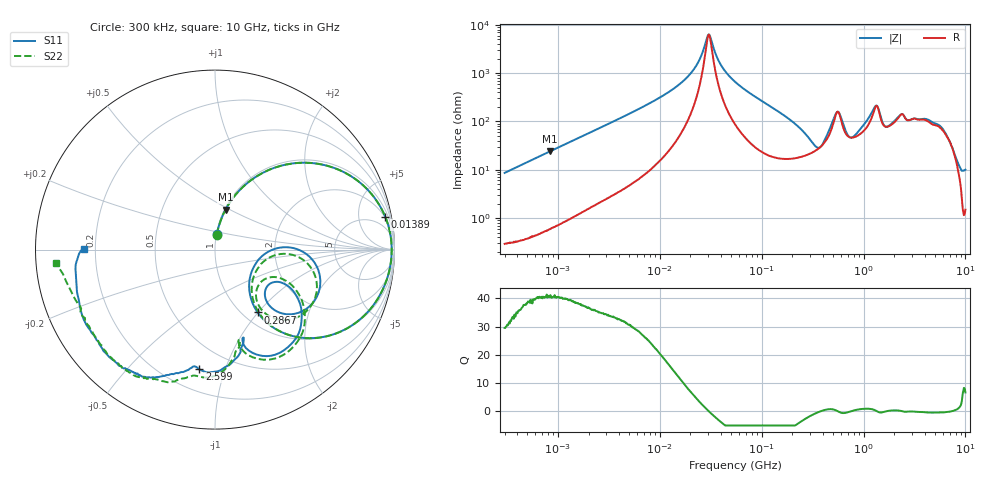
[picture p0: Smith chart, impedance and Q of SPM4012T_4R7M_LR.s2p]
! S-Parameter Data Generated by TDK Corporation
! Copyright(C) 2019 TDK Corporation.
! All Rights Reserved.
! TDK P/N: SPM4012T-4R7M-LR (Inductor)
! Property: L=4.7uH at 100kHz
! Size(LxWxT): 4.4x4.1x1.2mm
! Model Type: s2p (Touchstone File Format Version 1.0)
! Frequency: DC=Yes Start=0.3MHz Stop=10000MHz 802points Log-sweep
! Model Generated on Sep. 23, 2019
! Port Assignments:
!  1 ---@@@--- 2
! Applicable Conditions:
!  Temperature = 25 degC
!  DC Bias Current = 0 A
!  Small Signal Operation
! Terms and conditions regarding TDK Simulation Models
! (1)This simulation model is being provided solely for informational purposes. Please refer to the specifications of the products in terms of detailed characteristics of such products.
! (2)In no event shall TDK Corporation of any of its subsidiaries be liable for any loss or damage arising, directly or indirectly,
!  From any information contained in this simulation model, including, but not limited to loss or damages arising from any inaccuracies, omissions or errors in connection with such information.
! (3)Any and all copyrights on this simulation model are owned by TDK Corporation.
!  Duplication or redistribution of this simulation model without prior written permission from TDK Corporation is prohibited.
! (4)This simulation model is subject to any modification or change without any prior notice.
! (5)Neither TDK Corporation nor any of its subsidiaries shall make any warranty, express or implied,
!  Including but not limited to the correctness, implied warranties of merchantability and fitness for a particular purpose with respect to this simulation models.
! (6)The use of this simulation model shall be deemed to have consented to the terms and conditions hereof.
# Hz S MA R 50
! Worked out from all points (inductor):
!   801 points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, 300 kHz to 10 GHz, reference 50 ohm
!   read as one part in series: L = 4.57 uH near 318.3 kHz
!   highest Q = 40.6 at 832.9 kHz (marker M1), where L = 4.57 uH
!   self-resonance near 30.31 MHz
!   S11 on the Smith chart (normalised r, x): 300 kHz: 1.01, +0.17; 13.89 MHz: 2, +10; 286.7 MHz: 1.17, -0.99; 2.599 GHz: 0.34, -0.82; 10 GHz: 0.16, +0.00
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300000  0.08476 83.1  0.9935 -5.0  0.9935 -4.9  0.08438 83.1
832928  0.2309 75.2  0.9672 -13.4  0.9675 -13.4  0.2307 75.2
1713600  0.4349 62.6  0.8888 -25.8  0.8891 -25.8  0.4348 62.6
9671944  0.9353 17.8  0.3123 -69.5  0.3124 -69.5  0.9352 17.8
1.388558e7  0.9662 10.9  0.1981 -75.0  0.1982 -75.1  0.9661 10.9
2.189307e7  0.9825 3.6  0.07851 -75.7  0.07853 -75.8  0.9825 3.6
3.031424e7  0.9845 -1.1  0.01556 -1.5  0.01558 -1.5  0.9844 -1.1
3.955676e7  0.9812 -5.0  0.06466 69.9  0.06466 69.9  0.9812 -5.1
5.477226e7  0.9705 -10.3  0.1456 72.1  0.1457 72.1  0.9704 -10.4
1.630679e8  0.7765 -38.8  0.5447 44.4  0.5448 44.4  0.7769 -38.8
2.867479e8  0.4231 -55.8  0.7591 12.6  0.7593 12.6  0.4284 -55.2
3.126428e8  0.3529 -54.5  0.7734 6.5  0.7735 6.5  0.3613 -53.4
3.970454e8  0.2399 -19.5  0.7484 -12.9  0.7486 -12.9  0.2637 -21.2
5.497689e8  0.612 -16.4  0.3816 -21.5  0.3817 -21.5  0.6132 -22.6
7.318083e8  0.3939 -44.3  0.6514 -15.9  0.6515 -15.9  0.3535 -49.5
9.789263e8  0.4284 -26.3  0.5845 -44.7  0.5846 -44.7  0.3974 -23.6
1.24442e9  0.639 -41.5  0.3432 -60.2  0.3434 -60.2  0.6345 -37.9
1.418928e9  0.6604 -64.0  0.2952 -31.0  0.2954 -31.0  0.6923 -61.3
1.767019e9  0.521 -72.1  0.4506 -51.0  0.4507 -51.1  0.5173 -74.9
2.598782e9  0.6731 -97.5  0.276 -62.6  0.276 -62.6  0.7118 -97.5
5.849356e9  0.8374 -131.6  0.1798 -85.1  0.1799 -85.1  0.8374 -134.9
1e10  0.7272 179.8  0.1237 -124.2  0.1237 -124.4  0.8903 -175.3
